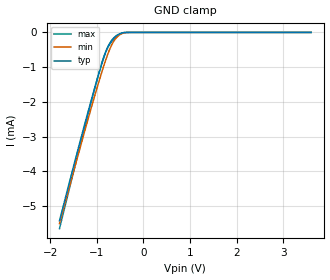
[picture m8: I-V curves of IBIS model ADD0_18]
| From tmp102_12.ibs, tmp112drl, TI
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|   ADD0_18   1.8V digital input Model
[Model] ADD0_18
Model_type   Input
| Signals   ADD0(4)
Vinl = 0.54
Vinh = 1.26
|   typ   min   max
|   (nom PVT)   (Fast PVT)   (slow PVT)
|Average
C_comp   5.8962090e-13  5.8962090e-13  5.9922750e-13
| Where   nom PVT is  Nominal Process, 1.8V, 27C
|   Fast PVT is Strong Process, 1.98V, -40C
|   Slow PVT is Weak Process, 1.62V, 125C
[Voltage Range]   1.8   1.62   1.98
[Temperature Range]   27   125   -40
|Ambient Temperature   27   125   -40
[Power Clamp Reference]   1.8   1.62   1.98
[GND Clamp Reference]   0   0   0
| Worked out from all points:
|   GND clamp passes 1 mA (typ) near -0.91 V on its own axis
[GND Clamp]
|   Voltage   I(typ)   I(min)   I(max)
-1.8V     -5.422mA   -5.502mA   -5.649mA
-1.266V   -2.675mA   -2.874mA   -2.767mA
-1.017V   -1.467mA   -1.695mA   -1.473mA
-894.6mV  -913.6uA   -1.15mA    -888.4uA
-816.7mV  -598.5uA   -825.2uA   -581.8uA
-750.5mV  -381uA     -577.7uA   -399.9uA
-714.6mV  -291.5uA   -458.9uA   -325.4uA
-648.4mV  -174uA     -278.8uA   -215.6uA
-544mV    -62.85uA   -107.4uA   -83.2uA
-426.2mV  -7.015uA   -17.92uA   -7.862uA
-287.6mV  -738.1nA   -782.2nA   -427nA
3.595V    0A         0A         0A
[POWER Clamp]
|   SCR cell for ESD function. Effects occurr above VDD x 2
|   Voltage   I(typ)   I(min)   I(max)
-1.8V     0A         0A         0A
0V        0A         0A         0A
3.6V      0A         0A         0A
